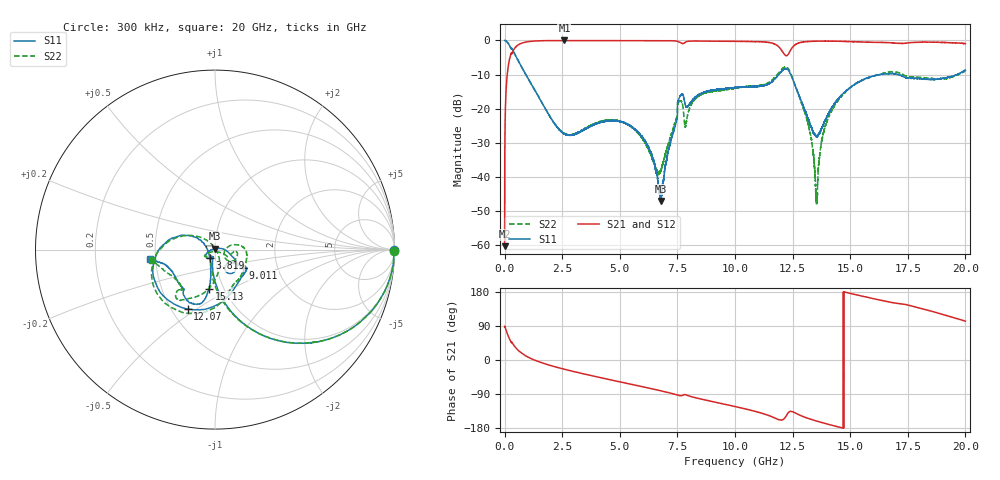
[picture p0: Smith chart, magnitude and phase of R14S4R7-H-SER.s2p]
!{R14S4R7}
!Johanson Technology Inc.
!www.johansontechnology.com
!Test Board Conditions:
!Substrate Type  RO4350B
!Substrate Thickness  20 mil
!Substrate Dk  3.66
!TL Type: GCPW
!TL Trace Width  36 mil
!TL Gap  12 mil
!Electrode orientation  Horizontal
!DUT TOPOLOGY	SERIES
!Mounting Pad LxW  26x36 mil
! Created Wed Nov 25 17:33:21 2020
! 2 Port Network Data from SP1.SP block
! freq  magS11  angS11  magS21  angS21  magS12  angS12  magS22  angS22
# khz S ma R 50
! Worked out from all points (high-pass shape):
!   20001 points, 300 kHz to 20 GHz, reference 50 ohm
!   highest |S21| = -0.01 dB at 2.596 GHz (marker M1); lowest = -60.4 dB at 300 kHz (marker M2)
!   |S21| within 3 dB of the highest: 367.5 MHz to 12.04 GHz (11.67 GHz wide, 188 % of centre); 12.4 GHz to end of sweep
!   lowest |S11| = -47.2 dB at 6.785 GHz (marker M3), VSWR 1.01, Z = 49.9 + j0.433 ohm
!   |S11| at or under -10 dB: 919.9 MHz to 11.9 GHz (10.98 GHz wide, 171 % of centre); 12.42 GHz to 16.32 GHz (3.897 GHz wide, 27.1 % of centre); 17.06 GHz to 19.63 GHz (2.571 GHz wide, 14 % of centre)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
!   |S22| runs from -48.2 to 0.0 dB; largest |S21 - S12| = 0.02
!   S11 on the Smith chart (normalised r, x): 300 kHz: open; 3.819 GHz: 0.94, -0.09; 9.011 GHz: 1.34, -0.28; 12.07 GHz: 0.60, -0.46; 15.13 GHz: 0.86, -0.39; 20 GHz: 0.47, -0.06
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300  0.9984 -0.2  0.0009532 86.6  0.0008507 86.4  0.9987 -0.3
112300  0.9486 -19.3  0.3123 70.6  0.313 70.6  0.9492 -19.3
307300  0.765 -42.3  0.6381 47.5  0.6398 47.5  0.7657 -42.1
990300  0.287 -80.7  0.9557 8.5  0.9555 8.5  0.287 -81.7
2596300  0.04248 -104.7  0.9986 -24.4  0.9967 -24.4  0.0428 -121.4
3334300  0.04631 -114.4  0.9959 -35.2  0.9961 -35.2  0.04755 -133.2
3819300  0.05665 -122.4  0.9958 -42.0  0.9962 -41.9  0.05842 -138.6
5655300  0.04906 -155.9  0.9953 -66.2  0.9946 -66.2  0.04835 -153.9
6667300  0.007465 156.1  0.9941 -79.8  0.9943 -79.8  0.0113 -97.9
6785300  0.004375 98.0  0.9954 -81.4  0.9944 -81.4  0.01242 -68.5
7600300  0.1493 -34.8  0.9404 -94.0  0.9409 -94.0  0.1293 -13.0
7874300  0.1063 -56.0  0.9547 -92.1  0.9541 -92.1  0.05935 1.9
9011300  0.1853 -32.6  0.9742 -109.6  0.9762 -109.6  0.178 -8.5
1.00003e7  0.2032 -29.8  0.9705 -122.8  0.97 -122.8  0.1991 -38.9
1.20693e7  0.364 -114.7  0.6799 -157.7  0.6852 -157.8  0.3902 -114.8
1.25683e7  0.2372 163.5  0.8428 -138.5  0.8417 -138.5  0.2401 165.9
1.33343e7  0.05117 164.0  0.9727 -157.3  0.9707 -157.2  0.03136 120.7
1.35473e7  0.03793 -162.3  0.9764 -161.3  0.975 -161.1  0.004665 11.1
1.39973e7  0.07723 -110.2  0.9759 -168.8  0.981 -168.8  0.0656 -66.6
1.51343e7  0.2195 -98.5  0.9565 173.8  0.9634 173.6  0.218 -98.9
1.66673e7  0.3232 -112.1  0.9286 153.5  0.9223 153.2  0.343 -124.5
2e7  0.3645 -171.7  0.8973 102.4  0.8964 102.7  0.3545 -170.9
